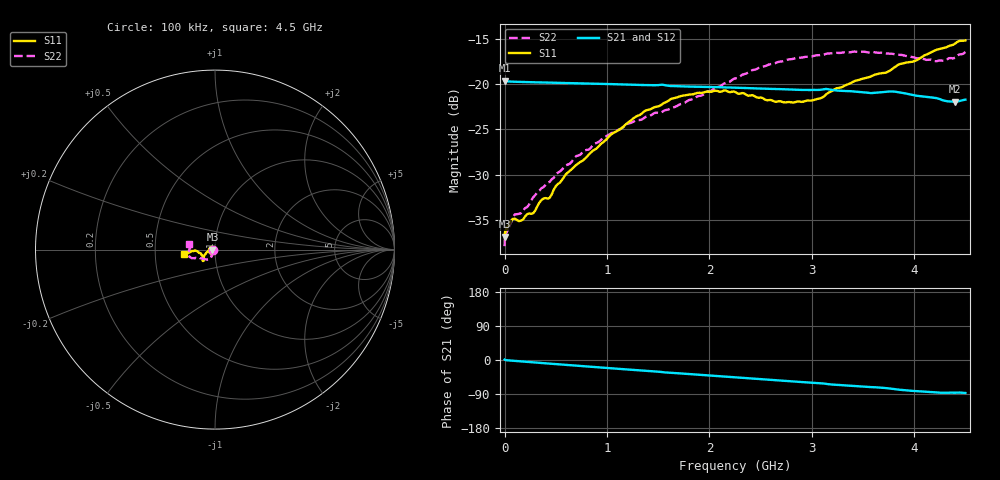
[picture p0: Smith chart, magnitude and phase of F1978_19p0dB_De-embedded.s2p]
! Integrated Device Technology
! Corporate Headquarters
! 6024 Silver Creek Valley Road
! San Jose, CA 95138  USA
! Phone:  1-408-284-8200
! Toll Free:  1-800-223-1366
! Webpage:  http://www.idt.com/
! Timing and RF Division
! 515 Groton Road, Suite 102
! Westford, MA 01886-6024
! Device:  F1978
! Description: 6-bit, 75 ohm, 0.5 dB Digital Step Attenuator
! Frequency:  5.0 MHz -  3.00 GHz
! Package:  4x4 mm QFN Plastic Package: 20 pin
! Ports:  2 RF, 11 DC
!  Pin  1  = D5 (16 dB)
!  Pin  2  = RF1  =  Port 1
!  Pin  3  = Serial Data In (DATA)
!  Pin  4  = Serial Clock (CLK)
!  Pin  5  = Serial Latch Enable (LE)
!  Pin  6  = VDD
!  Pin  7  = NC
!  Pin  8  = NC
!  Pin  9  = NC
!  Pin 10  = GND
!  Pin 11  = GND
!  Pin 12  = NC
!  Pin 13  = VMODE
!  Pin 14  = RF2  =  Port 2
!  Pin 15  = D4 (8 dB)
!  Pin 16  = D3 (4 dB)
!  Pin 17  = D2 (2 dB)
!  Pin 18  = NC
!  Pin 19  = D1 (1 dB)
!  Pin 20  = D0 (0.5 dB)
! State:  38
! Atten State:  19.0 dB
! Voltage:  +3.30 Volts
! Current:  0.590 mA
! Data:  The device was measured on a F1975 evaluation board which has
!  individual transmission lines to the RF pins.  Data was collected
!  using a calibrated network analyzer.  The evaluation board was
!  de-embedded using Automatic Fixture Removal (AFR).
!  The reference plane is the edge of the package pin.
! Misc:
!  Action Tracker AT0416
! Date Measured:  2018-02-08
! Date:  2018-03-26  MJV
! Note:
!  Integrated Device Technology supplies this data as a sample of measured
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# GHz S dB R 75
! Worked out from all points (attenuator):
!   291 points, 100 kHz to 4.5 GHz, reference 75 ohm
!   highest |S21| = -19.63 dB at 100 kHz (marker M1); lowest = -21.9 dB at 4.4 GHz (marker M2)
!   lowest |S11| = -36.8 dB at 300 kHz (marker M3), VSWR 1.03, Z = 72.9 - j0.0299 ohm
!   |S11| at or under -10 dB: start of sweep to end of sweep
!   |S22| runs from -37.9 to -16.4 dB; largest |S21 - S12| = 0.00016
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0.0001  -36.82 179.8  -19.63 1.2  -19.63 1.2  -37.87 -178.0
0.0003  -36.83 -179.2  -19.63 1.1  -19.64 1.1  -37.68 -178.0
0.003  -36.39 -177.9  -19.67 0.7  -19.67 0.7  -36.94 -176.1
0.013  -36.11 -177.9  -19.70 -0.5  -19.69 -0.5  -36.45 -173.1
0.1  -34.83 -174.8  -19.74 -2.4  -19.73 -2.4  -34.37 -155.1
0.16  -35.04 -176.4  -19.76 -3.7  -19.76 -3.7  -34.24 -145.3
0.28  -34.23 -179.0  -19.79 -6.2  -19.79 -6.2  -32.47 -135.1
0.36  -32.80 -178.9  -19.82 -7.9  -19.81 -7.9  -31.47 -127.4
0.44  -32.54 -178.2  -19.84 -9.5  -19.83 -9.5  -30.78 -122.1
0.6  -29.92 -174.4  -19.88 -12.8  -19.88 -12.8  -28.94 -118.8
0.76  -28.46 -167.3  -19.92 -16.1  -19.92 -16.1  -27.53 -117.5
1.26  -23.76 -152.4  -20.07 -26.2  -20.07 -26.2  -24.14 -120.4
1.52  -22.37 -144.7  -20.08 -31.3  -20.08 -31.2  -23.17 -127.8
1.88  -20.97 -138.2  -20.29 -38.5  -20.28 -38.5  -21.36 -142.9
2.26  -20.92 -137.2  -20.39 -45.9  -20.39 -45.9  -19.35 -154.5
2.64  -21.94 -147.7  -20.53 -53.3  -20.53 -53.3  -17.70 -158.6
3.02  -21.76 -164.3  -20.64 -60.3  -20.63 -60.3  -16.89 -162.2
3.42  -19.65 -175.7  -20.82 -69.0  -20.82 -69.0  -16.41 -168.7
3.76  -18.53 -176.0  -20.81 -75.2  -20.81 -75.2  -16.64 -175.8
4.2  -16.30 -172.9  -21.51 -85.1  -21.51 -85.1  -17.47 171.8
4.4  -15.53 -170.8  -21.95 -86.3  -21.94 -86.3  -17.07 168.5
4.5  -15.19 -172.5  -21.71 -87.1  -21.71 -87.1  -16.46 167.1
